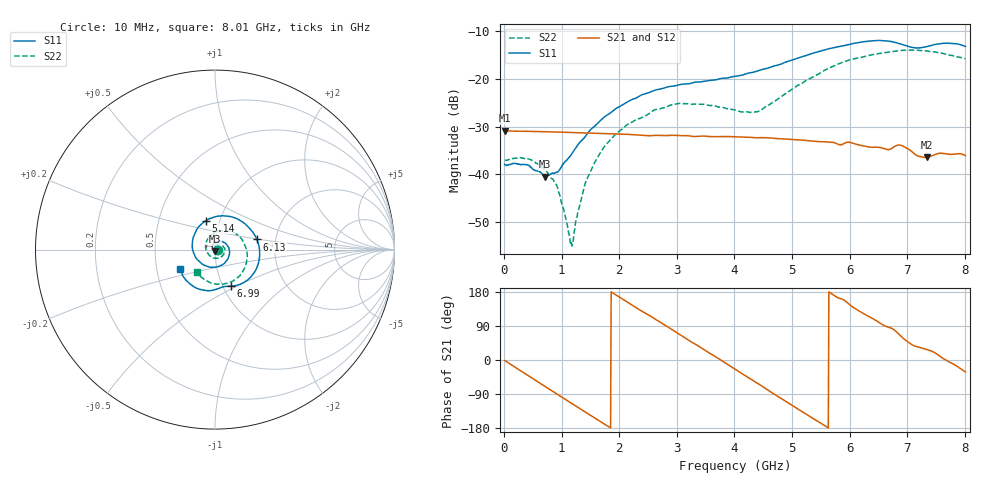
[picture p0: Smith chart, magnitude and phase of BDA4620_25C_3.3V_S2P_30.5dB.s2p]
!Agilent Technologies,E5071B,MY42404982,A.09.10
!Date: Wed May 06 08:55:30 2026
!Data & Calibration Information:
!Freq	S11:SOLT2(ON)	S21:SOLT2(ON)	S12:SOLT2(ON)	S22:SOLT2(ON)
# Hz S RI R 50
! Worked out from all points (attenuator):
!   801 points, 10 MHz to 8.01 GHz, reference 50 ohm
!   highest |S21| = -30.86 dB at 20 MHz (marker M1); lowest = -36.4 dB at 7.34 GHz (marker M2)
!   lowest |S11| = -40.5 dB at 710 MHz (marker M3), VSWR 1.02, Z = 49.9 - j0.937 ohm
!   |S11| at or under -10 dB: start of sweep to end of sweep
!   |S22| runs from -55.1 to -13.9 dB; largest |S21 - S12| = 0.00016
!   S11 on the Smith chart (normalised r, x): 10 MHz: 1.03, -0.00; 5.14 GHz: 0.86, +0.29; 6.13 GHz: 1.60, +0.19; 6.99 GHz: 1.10, -0.47; 8.01 GHz: 0.66, -0.15
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1e7  0.0127 -0.000775  0.0286 -0.000592  0.0287 -0.00059  0.014 -0.000463
2e7  0.0125 -0.00078  0.0286 -0.00104  0.0287 -0.00117  0.014 -0.000368
4.4e8  0.0085 -0.0089  0.0206 -0.0193  0.0206 -0.0194  0.0135 -0.00509
7.1e8  -0.000734 -0.00939  0.00978 -0.0262  0.00981 -0.0263  0.00869 -0.00712
9.3e8  -0.00913 -0.00524  -0.000414 -0.0278  -0.000452 -0.0278  0.00355 -0.00627
1.16e9  -0.0151 0.0052  -0.0108 -0.0253  -0.0109 -0.0253  -0.0014 -0.00118
1.2e9  -0.0156 0.00742  -0.0125 -0.0245  -0.0125 -0.0245  -0.002 1.17e-05
1.35e9  -0.0159 0.0163  -0.0181 -0.0204  -0.0181 -0.0204  -0.0035 0.00456
1.53e9  -0.0119 0.0281  -0.0231 -0.0141  -0.0231 -0.0141  -0.00337 0.0111
1.77e9  0.00114 0.041  -0.0264 -0.0039  -0.0265 -0.00388  0.000646 0.0203
2.14e9  0.0343 0.0461  -0.0234 0.012  -0.0234 0.012  0.0164 0.0289
2.68e9  0.0777 0.00723  -0.00559 0.0249  -0.00557 0.025  0.0441 0.0196
3.08e9  0.0741 -0.0475  0.011 0.023  0.0111 0.023  0.0551 -0.00702
4.01e9  -0.0684 -0.0824  0.0226 -0.0101  0.0226 -0.0102  -0.0101 -0.0463
4.43e9  -0.1232 -0.00536  0.0105 -0.0218  0.0105 -0.0219  -0.0445 -0.0117
5.14e9  -0.0509 0.1619  -0.0156 -0.0167  -0.0157 -0.0168  -0.0123 0.0872
5.35e9  0.0112 0.1856  -0.0199 -0.0102  -0.0199 -0.0102  0.0229 0.1016
6.13e9  0.2339 0.0563  -0.0139 0.0151  -0.0139 0.0152  0.1618 0.0359
6.68e9  0.1917 -0.1605  0.00123 0.0181  0.00127 0.0182  0.1697 -0.0897
6.99e9  0.0909 -0.2034  0.012 0.0145  0.0121 0.0145  0.1262 -0.1564
7.34e9  0.0144 -0.2188  0.0133 0.00701  0.0134 0.00703  0.043 -0.1924
8.01e9  -0.1924 -0.1069  0.0135 -0.00827  0.0135 -0.0083  -0.1013 -0.1273
